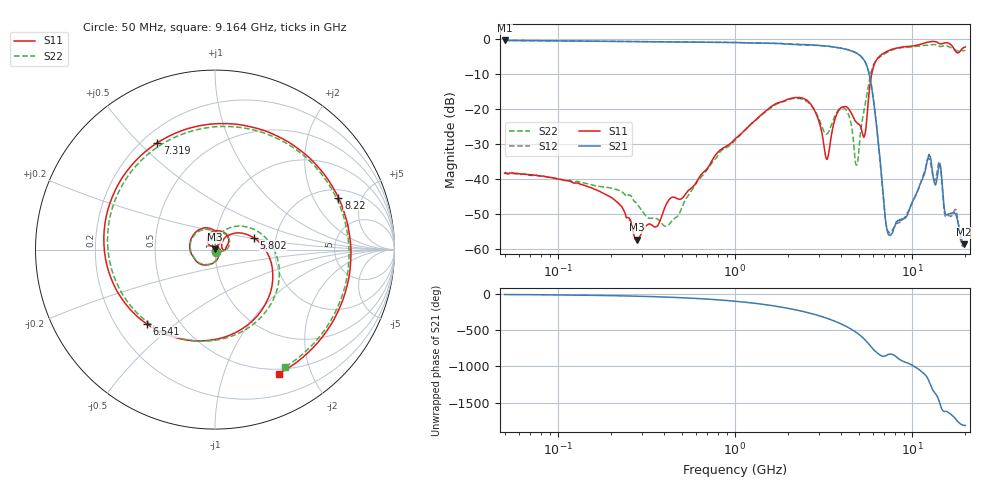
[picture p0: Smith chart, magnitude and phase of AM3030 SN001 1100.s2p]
# Hz S DB R 50
!freq MagS11 AngS11 MagS21 AngS21 MagS12 AngS12 MagS22 AngS22
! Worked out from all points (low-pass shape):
!   1601 points, 50 MHz to 20.05 GHz, reference 50 ohm
!   highest |S21| = -0.40 dB at 50 MHz (marker M1); lowest = -58.7 dB at 19.6 GHz (marker M2)
!   |S21| within 3 dB of the highest: start of sweep to 4.559 GHz
!   lowest |S11| = -57.4 dB at 280.1 MHz (marker M3), VSWR 1.00, Z = 49.9 + j0.0558 ohm
!   |S11| at or under -10 dB: start of sweep to 5.928 GHz
!   |S22| runs from -53.6 to -1.6 dB; largest |S21 - S12| = 0.018
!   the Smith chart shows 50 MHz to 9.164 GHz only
!   S11 on the Smith chart (normalised r, x): 50 MHz: 1.01, -0.02; 5.802 GHz: 1.53, +0.21; 6.541 GHz: 0.33, -0.40; 7.319 GHz: 0.26, +0.57; 8.22 GHz: 2.44, +3.19; 9.164 GHz: 0.44, -1.55
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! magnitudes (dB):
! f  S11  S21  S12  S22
! 50 MHz  -38.4  -0.4  -0.4  -38.1
! 135.9 MHz  -41.6  -0.6  -0.6  -41.0
! 280.1 MHz  -57.4  -0.7  -0.7  -47.2
! 369.6 MHz  -53.1  -0.8  -0.8  -51.7
! 1.005 GHz  -28.5  -1.0  -1.0  -28.9
! 2.722 GHz  -19.1  -1.7  -1.8  -19.2
! 3.308 GHz  -34.4  -2.0  -2.0  -27.2
! 4.188 GHz  -19.3  -2.9  -2.8  -20.0
! 4.865 GHz  -23.9  -4.0  -4.0  -36.1
! 5.383 GHz  -27.9  -6.1  -6.1  -19.9
! 5.802 GHz  -12.9  -11.2  -11.1  -10.7
! 6.541 GHz  -5.0  -32.1  -32.5  -5.2
! 7.319 GHz  -3.4  -55.6  -55.0  -3.7
! 7.402 GHz  -3.3  -56.1  -55.3  -3.5
! 8.22 GHz  -2.5  -52.3  -52.7  -2.7
! 9.164 GHz  -2.2  -51.2  -50.8  -2.4
! 12.51 GHz  -0.8  -33.1  -34.2  -1.8
! 14.31 GHz  -1.3  -35.9  -35.1  -2.1
! 15.48 GHz  -1.0  -50.1  -50.8  -1.9
! 17.65 GHz  -3.5  -50.1  -48.7  -3.2
! 19.6 GHz  -2.4  -58.7  -58.9  -3.3
! 20.05 GHz  -2.3  -58.5  -58.2  -3.2
